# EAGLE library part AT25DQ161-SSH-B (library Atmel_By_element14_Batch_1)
SPI Serial EEPROM
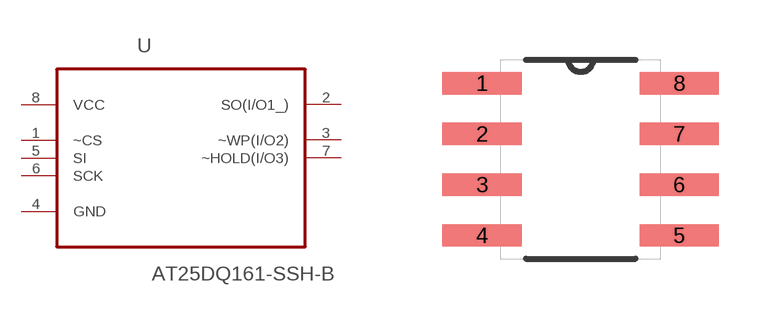
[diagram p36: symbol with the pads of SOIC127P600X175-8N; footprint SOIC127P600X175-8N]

Designator prefix U

## AT25DQ161-SSH-B (MPN: AT25DQ161-SSH-B; OC_FARNELL: 1841585; OC_NEWARK: 12T1351; PACKAGE: SOIC-8; SUPPLIER: Atmel)  [SOIC127P600X175-8N]
1  ~CS  in
2  SO(I/O1_)
3  ~WP(I/O2)
4  GND  pas
5  SI  in
6  SCK  in
7  ~HOLD(I/O3)
8  VCC  pwr

## Footprint SOIC127P600X175-8N (pad centres in mm)
smd 1.981 x 0.559: 1 -2.464,1.905; 2 -2.464,0.635; 3 -2.464,-0.635; 4 -2.464,-1.905; 5 2.464,-1.905; 6 2.464,-0.635; 7 2.464,0.635; 8 2.464,1.905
